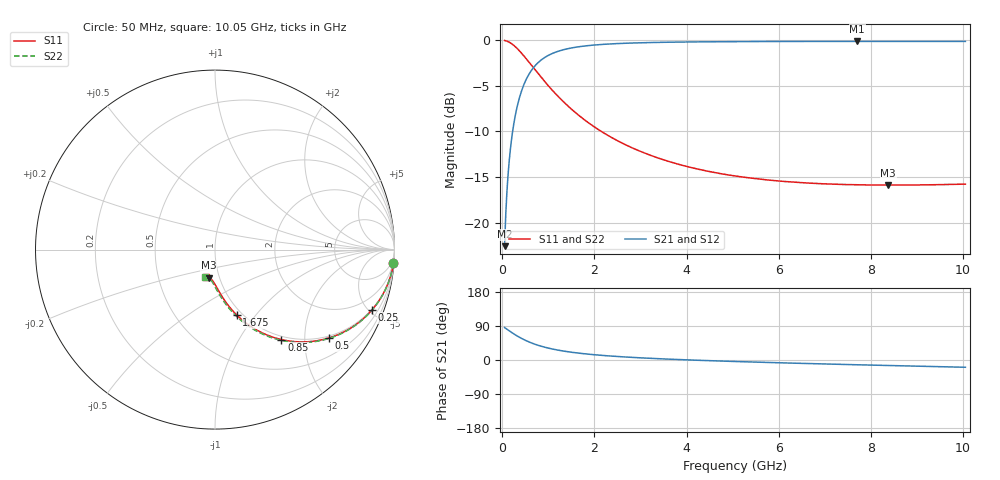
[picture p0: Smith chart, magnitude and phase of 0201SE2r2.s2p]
! AVX Thin Film Operation		Date: August 2001
! Description: Accu-P® Series, Thin Film, SMD, RF Capacitor
! Part Number: 02013J2R2ABW
! 50 MHz  -  10.05 GHz
! Serial Measurements
# mhz S db R 50
!	S11		S21		S12		S22
!	dB	Phase	dB	Phase	dB	Phase	dB	Phase
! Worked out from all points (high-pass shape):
!   401 points, 50 MHz to 10.05 GHz, reference 50 ohm
!   highest |S21| = -0.12 dB at 7.7 GHz (marker M1); lowest = -22.6 dB at 50 MHz (marker M2)
!   |S21| within 3 dB of the highest: 658 MHz to end of sweep
!   lowest |S11| = -15.9 dB at 8.375 GHz (marker M3), VSWR 1.38, Z = 44.4 - j14.3 ohm
!   |S11| at or under -10 dB: 2.15 GHz to end of sweep
!   |S22| runs from -15.9 to 0.0 dB; largest |S21 - S12| = 0
!   S11 on the Smith chart (normalised r, x): 50 MHz: 1, -26; 250 MHz: 0.95, -5.21; 500 MHz: 0.94, -2.61; 850 MHz: 0.94, -1.55; 1.675 GHz: 0.94, -0.81; 10.05 GHz: 0.87, -0.28
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50  -0.02 -4.4  -22.57 85.6  -22.57 85.6  -0.02 -4.4
75  -0.05 -6.6  -19.08 83.4  -19.08 83.4  -0.05 -6.6
125  -0.15 -10.9  -14.74 79.1  -14.74 79.1  -0.15 -11.0
150  -0.21 -13.0  -13.22 77.0  -13.22 77.0  -0.21 -13.1
200  -0.37 -17.1  -10.88 72.8  -10.88 72.8  -0.37 -17.2
250  -0.57 -21.1  -9.14 68.8  -9.14 68.8  -0.57 -21.2
350  -1.04 -28.4  -6.71 61.5  -6.71 61.5  -1.04 -28.6
500  -1.91 -37.9  -4.49 51.9  -4.49 51.9  -1.91 -38.2
650  -2.85 -45.6  -3.18 44.2  -3.18 44.2  -2.85 -46.0
850  -4.11 -53.6  -2.14 36.1  -2.14 36.1  -4.11 -54.1
1025  -5.14 -59.0  -1.59 30.7  -1.59 30.7  -5.14 -59.6
1200  -6.10 -63.3  -1.23 26.3  -1.23 26.3  -6.10 -64.0
1675  -8.29 -71.5  -0.70 17.9  -0.70 17.9  -8.29 -72.6
1725  -8.50 -72.2  -0.67 17.2  -0.67 17.2  -8.49 -73.3
2500  -11.01 -79.9  -0.36 9.2  -0.36 9.2  -11.01 -81.4
3400  -12.94 -85.6  -0.23 3.4  -0.23 3.4  -12.94 -87.4
5050  -14.88 -92.5  -0.15 -4.0  -0.15 -4.0  -14.88 -94.9
6725  -15.68 -98.0  -0.13 -9.6  -0.13 -9.6  -15.68 -100.5
7700  -15.84 -100.9  -0.12 -12.6  -0.12 -12.6  -15.85 -103.4
8375  -15.88 -102.8  -0.12 -14.5  -0.12 -14.5  -15.88 -105.3
8400  -15.88 -102.9  -0.12 -14.6  -0.12 -14.6  -15.88 -105.4
10050  -15.77 -107.5  -0.13 -19.2  -0.13 -19.2  -15.77 -109.9
